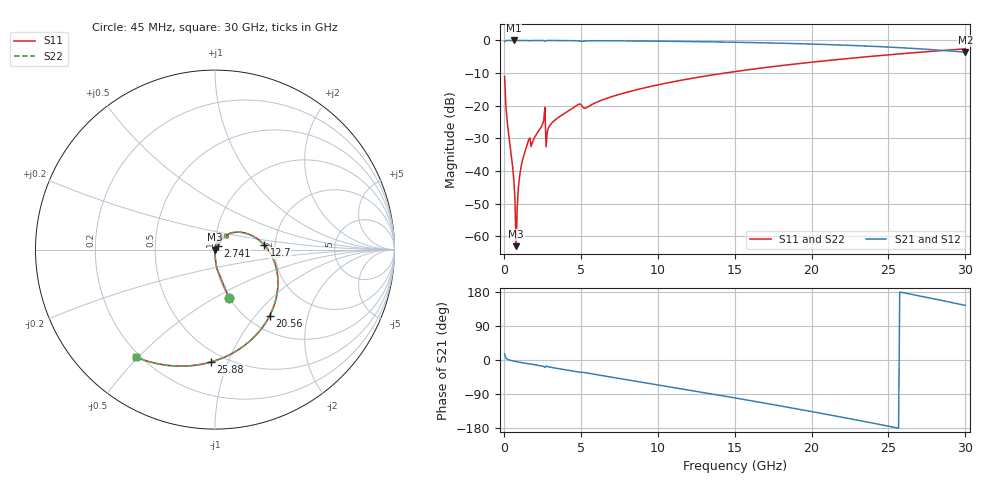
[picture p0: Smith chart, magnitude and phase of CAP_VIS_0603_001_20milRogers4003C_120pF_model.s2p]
! S-parameter model data by Modelithics Inc.  support@modelithics.com  813-866-6335  Tampa FL USA
! S-Parameter data specifications:
! Substrate: 20-mil Rogers 4003C, substrate thickness, H=0.508mm, Dielectric constant, Er=3.75
! PCB Mounting Pad Footprint: Pad width, PadW=0.90mm , Pad length, PadL=1.00mm , Pad gap, PadG (edge-to-edge)=1.00mm , Reference planes=3.0mm apart
! Created Wed Nov 18 13:31:47 2015
# hz S ma R 50
! 2 Port Network Data from SP1.SP block
! freq  magS11  angS11  magS21  angS21  magS12  angS12  magS22  angS22
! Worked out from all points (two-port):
!   401 points, 45 MHz to 30 GHz, reference 50 ohm
!   highest |S21| = -0.01 dB at 644.1 MHz (marker M1); lowest = -3.6 dB at 30 GHz (marker M2)
!   |S21| within 3 dB of the highest: start of sweep to 28.38 GHz
!   lowest |S11| = -63.0 dB at 793.9 MHz (marker M3), VSWR 1.00, Z = 50.1 - j0.0301 ohm
!   |S11| at or under -10 dB: start of sweep to 14.34 GHz
!   |S22| runs from -63.0 to -2.6 dB; largest |S21 - S12| = 0
!   S11 on the Smith chart (normalised r, x): 45 MHz: 1.00, -0.59; 2.741 GHz: 1.03, +0.04; 12.7 GHz: 1.75, +0.10; 20.56 GHz: 1.24, -1.19; 25.88 GHz: 0.42, -0.87; 30 GHz: 0.18, -0.49
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4.5e7  0.2813 -73.9  0.9594 16.1  0.9594 16.1  0.2813 -73.9
5.692125e8  0.01154 -89.6  0.9993 -2.4  0.9993 -2.4  0.01154 -89.6
6.441e8  0.007294 -88.3  0.9993 -3.0  0.9993 -3.0  0.007294 -88.3
7.93875e8  0.0007055 -25.2  0.9993 -4.2  0.9993 -4.2  0.0007055 -25.2
9.4365e8  0.00563 77.3  0.9992 -5.4  0.9992 -5.4  0.00563 77.3
1.018538e9  0.008272 78.9  0.9991 -5.9  0.9991 -5.9  0.008272 78.9
1.168312e9  0.01326 79.4  0.999 -7.0  0.999 -7.0  0.01326 79.4
1.54275e9  0.02628 76.5  0.9978 -9.8  0.9978 -9.8  0.02628 76.5
1.917188e9  0.03003 74.6  0.9976 -12.0  0.9976 -12.0  0.03003 74.6
2.516288e9  0.05229 71.4  0.9965 -16.5  0.9965 -16.5  0.05229 71.4
2.74095e9  0.02343 52.9  0.9911 -15.9  0.9911 -15.9  0.02343 52.9
2.890725e9  0.0454 69.8  0.997 -18.1  0.997 -18.1  0.0454 69.8
3.414938e9  0.06288 66.8  0.9963 -21.9  0.9963 -21.9  0.06288 66.8
5.062462e9  0.1011 43.3  0.9702 -32.7  0.9702 -32.7  0.1011 43.3
1.007992e10  0.2105 23.4  0.9743 -66.0  0.9743 -66.0  0.2105 23.4
1.270099e10  0.2749 5.6  0.9577 -83.9  0.9577 -83.9  0.2749 5.6
1.50225e10  0.3336 -10.5  0.9384 -100.1  0.9384 -100.1  0.3336 -10.5
2.003996e10  0.4651 -46.8  0.8797 -136.4  0.8797 -136.4  0.4651 -46.8
2.056418e10  0.4792 -50.7  0.872 -140.3  0.872 -140.3  0.4792 -50.7
2.505742e10  0.6034 -85.4  0.7903 -175.1  0.7903 -175.1  0.6034 -85.4
2.588119e10  0.6267 -92.1  0.7717 178.3  0.7717 178.3  0.6267 -92.1
3e10  0.7433 -126.2  0.6594 144.2  0.6594 144.2  0.7433 -126.2
